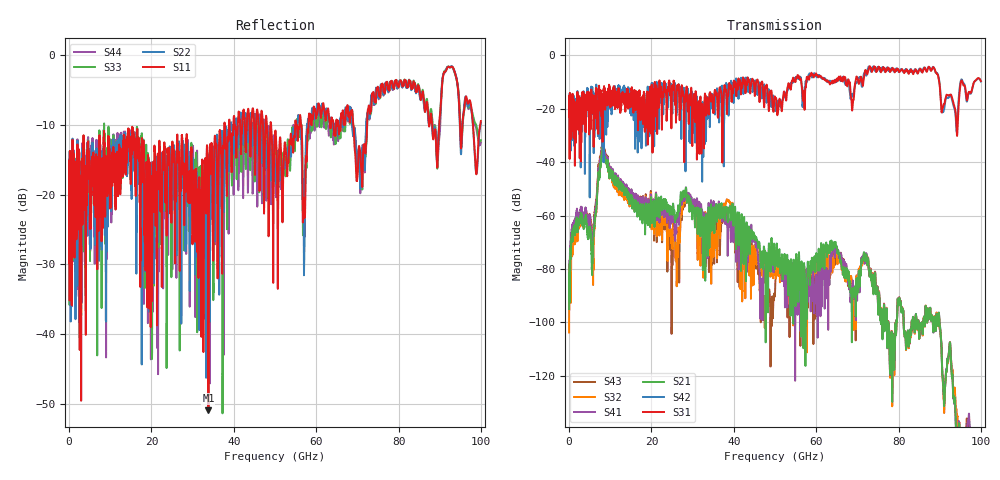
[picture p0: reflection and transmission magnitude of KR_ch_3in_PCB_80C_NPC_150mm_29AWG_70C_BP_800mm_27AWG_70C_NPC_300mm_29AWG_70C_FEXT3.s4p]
# GHz S RI R 45
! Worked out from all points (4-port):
!   4000 points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, 25 MHz to 100 GHz, reference 45 ohm
!   strongest paths, dB at 25 MHz, 25.02 GHz, 50.02 GHz, 75.03 GHz, 100 GHz:
!     S31: -20.7, -12.5, -15.6, -4.9, -9.6
!     S42: -20.7, -17.7, -18.0, -4.4, -9.7
!     S21: -95.0, -58.5, -77.7, -95.4, -159.8
!     S41: -94.5, -61.7, -77.4, -95.3, -154.9
!     S32: -103.7, -68.9, -78.5, -95.1, -162.0
!     S43: -95.0, -75.7, -88.6, -94.9, -169.2
!   lowest |S11| = -50.9 dB at 33.85 GHz (marker M1), VSWR 1.01, Z = 45.2 + j0.102 ohm
!   |S11| at or under -10 dB: start of sweep to 37.71 GHz; 49.07 GHz to 54.91 GHz (5.84 GHz wide, 11.2 % of centre); 68.98 GHz to 72.37 GHz (3.391 GHz wide, 4.8 % of centre)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
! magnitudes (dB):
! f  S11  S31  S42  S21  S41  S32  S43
! 25 MHz  -16.4  -20.7  -20.7  -95.0  -94.5  -103.7  -95.0
! 5.775 GHz  -14.6  -16.4  -16.4  -75.1  -68.7  -77.7  -68.2
! 8.225 GHz  -21.4  -31.4  -21.3  -34.4  -32.8  -33.0  -31.7
! 26.3 GHz  -11.4  -11.3  -18.6  -60.1  -62.1  -72.7  -74.9
! 28.62 GHz  -12.7  -12.6  -14.3  -54.2  -54.1  -54.3  -54.5
! 33.85 GHz  -50.9  -21.8  -23.4  -58.1  -55.8  -64.0  -58.4
! 100 GHz  -9.5  -9.6  -9.7  -159.8  -154.9  -162.0  -169.2
